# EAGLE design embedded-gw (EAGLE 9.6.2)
AUTHOR: Neal Jackson; REV: B; TITLE: Embedded GW

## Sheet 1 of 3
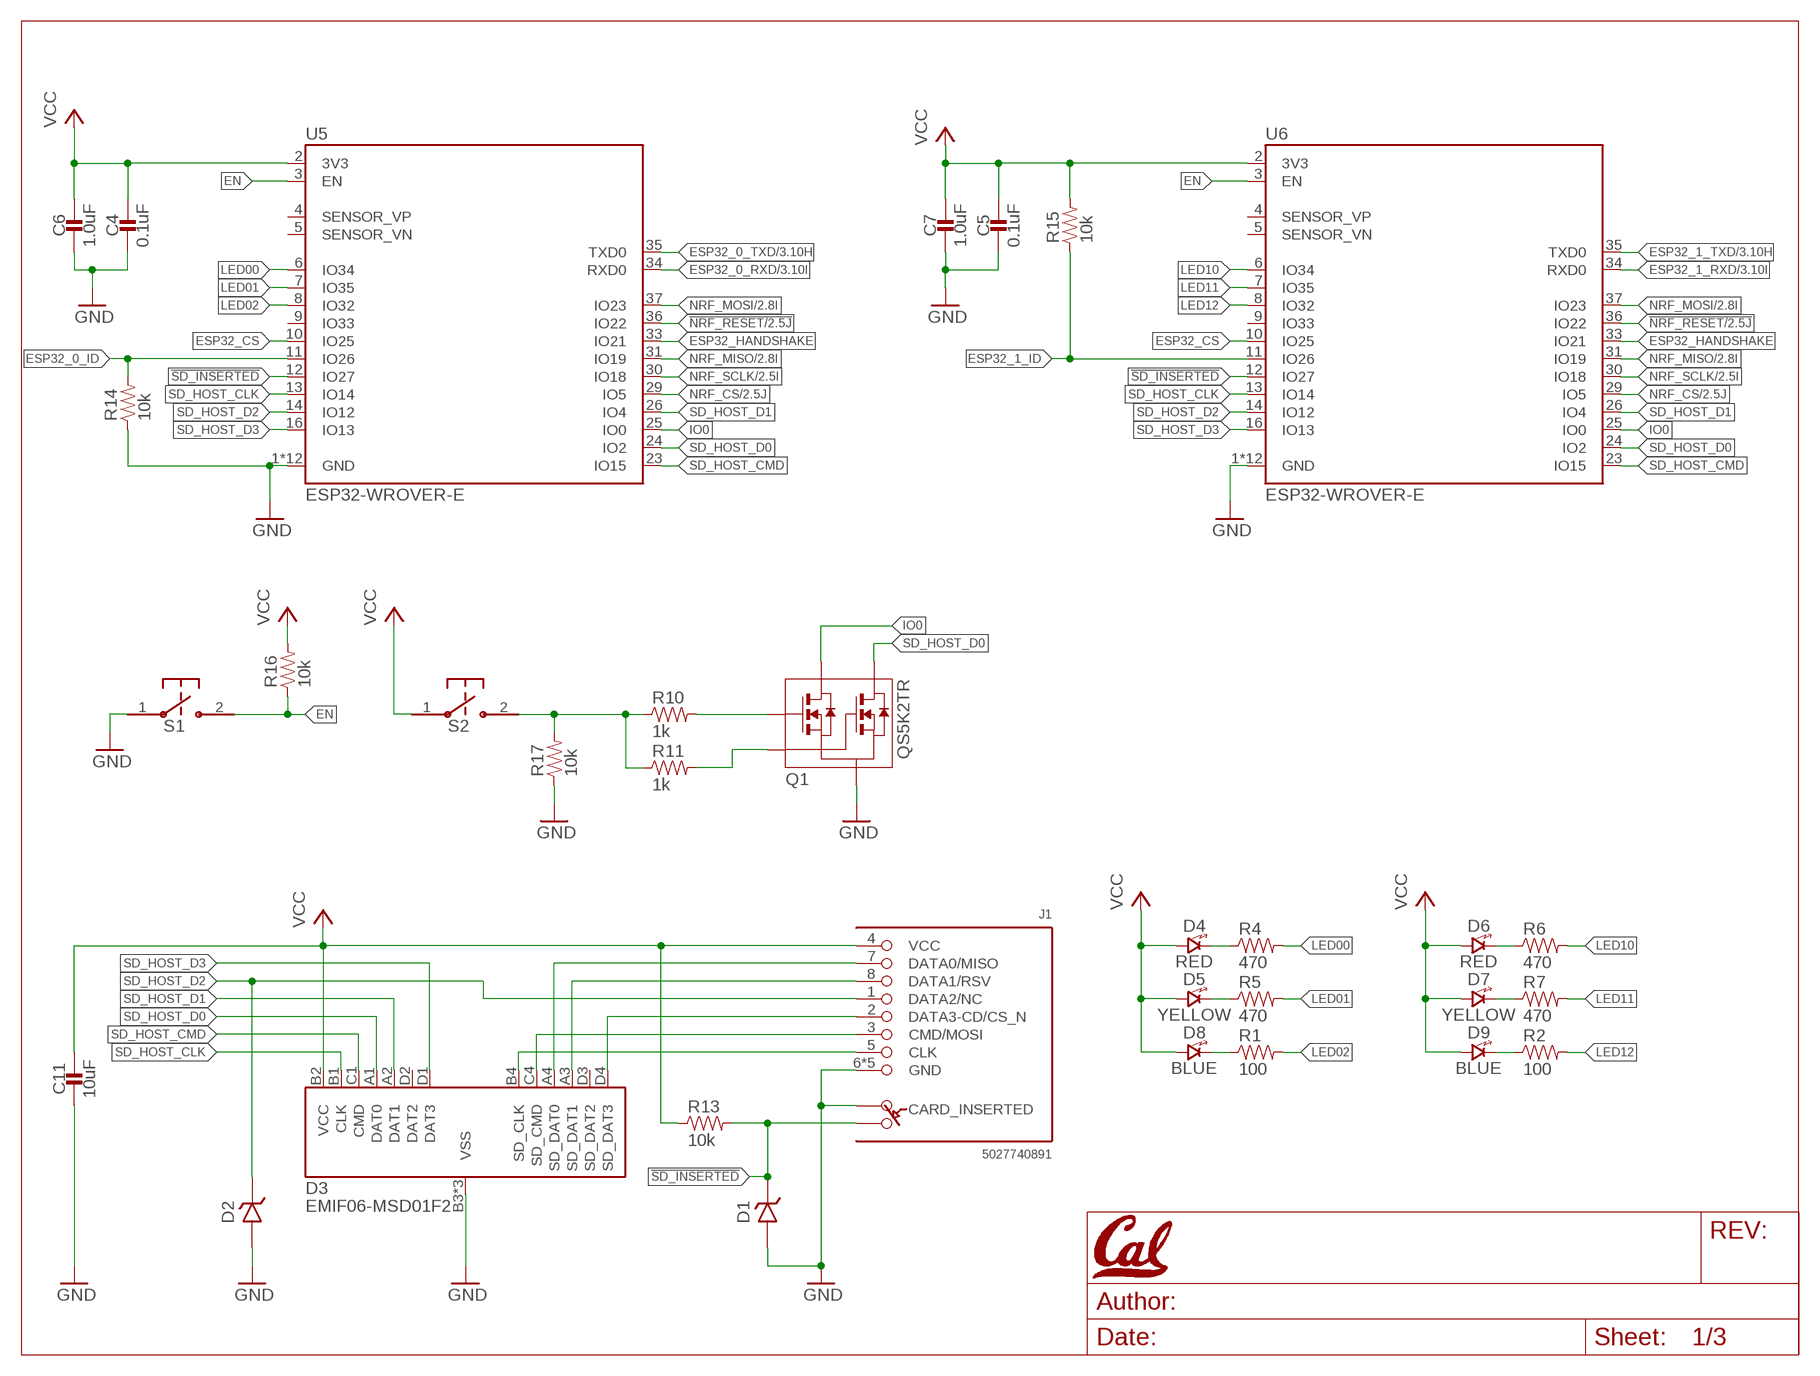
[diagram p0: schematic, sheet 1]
U$1 (LETTER_L_CAL): HEIGHT: 8.5in; WIDTH: 11in

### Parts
C4  0.1uF  CAPACITOR0402_CAP  [0402_CAP]
C5  0.1uF  CAPACITOR0402_CAP  [0402_CAP]
C6  1.0uF  CAPACITOR0402_CAP  [0402_CAP]
C7  1.0uF  CAPACITOR0402_CAP  [0402_CAP]
C11  10uF  CAPACITOR0805_CAP  [0805_CAP]
D1  DIODE_ZENER0201  [0201_DIODE]
D2  DIODE_ZENER0201  [0201_DIODE]
D3  EMIF06-MSD01F2  [BGA16C50P4X4_192X192X65N]
D4  RED  LED0603  [LED-0603]
D5  YELLOW  LED0603  [LED-0603]
D6  RED  LED0603  [LED-0603]
D7  YELLOW  LED0603  [LED-0603]
D8  BLUE  LED0603  [LED-0603]
D9  BLUE  LED0603  [LED-0603]
J1  5027740891  [5027740891]
Q1  QS5K2TR  [SOT95P280X100-5N]
R1  100  RESISTOR0402_RES  [0402_RES]
R2  100  RESISTOR0402_RES  [0402_RES]
R4  470  RESISTOR0402_RES  [0402_RES]
R5  470  RESISTOR0402_RES  [0402_RES]
R6  470  RESISTOR0402_RES  [0402_RES]
R7  470  RESISTOR0402_RES  [0402_RES]
R10  1k  RESISTOR0402_RES  [0402_RES]
R11  1k  RESISTOR0402_RES  [0402_RES]
R13  10k  RESISTOR0402_RES  [0402_RES]
R14  10k  RESISTOR0402_RES  [0402_RES]
R15  10k  RESISTOR0402_RES  [0402_RES]
R16  10k  RESISTOR0402_RES  [0402_RES]
R17  10k  RESISTOR0402_RES  [0402_RES]
S1  B3U-1000P  [B3U-1000P]
S2  B3U-1000P  [B3U-1000P]
U5  ESP32-WROVER-E  [ESP32-WROVER-E]
U6  ESP32-WROVER-E  [ESP32-WROVER-E]

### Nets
!NRF_RESET: U5.36(IO22) U6.36(IO22) ; also sheet 2
!SD_INSERTED: D1.P$1(CATHODE) J1.SWITCH(B) R13.2 U5.12(IO27) U6.12(IO27)
EN: R16.1 S1.2 U5.3(EN) U6.3(EN)
ESP32_0_ID: R14.2 U5.11(IO26)
ESP32_0_RXD: U5.34(RXD0) ; also sheet 3
ESP32_0_TXD: U5.35(TXD0) ; also sheet 3
ESP32_1_ID: R15.1 U6.11(IO26)
ESP32_1_RXD: U6.34(RXD0) ; also sheet 3
ESP32_1_TXD: U6.35(TXD0) ; also sheet 3
ESP32_CS: U5.10(IO25) U6.10(IO25)
ESP32_HANDSHAKE: U5.33(IO21) U6.33(IO21)
GND: C4.2 C5.2 C6.2 C7.2 C11.P$2 D1.P$2(ANODE) D2.P$2(ANODE) D3.B3(VSS) D3.C2(VSS) D3.C3(VSS) J1.6(GND) J1.DETECT(A) J1.GND1(GND) J1.GND2(GND) J1.GND3(GND) J1.GND4(GND) Q1.2(S) R14.1 R17.1 S1.1 U5.1(GND) U5.15(GND) U5.38(GND) U5.GND1(GND) U5.GND2(GND) U5.GND3(GND) U5.GND4(GND) U5.GND5(GND) U5.GND6(GND) U5.GND7(GND) U5.GND8(GND) U5.GND9(GND) U6.1(GND) U6.15(GND) U6.38(GND) U6.GND1(GND) U6.GND2(GND) U6.GND3(GND) U6.GND4(GND) U6.GND5(GND) U6.GND6(GND) U6.GND7(GND) U6.GND8(GND) U6.GND9(GND) ; also sheet 2,3
IO0: Q1.5(D1) U5.25(IO0) U6.25(IO0)
LED00: R4.2 U5.6(IO34)
LED01: R5.2 U5.7(IO35)
LED02: R1.2 U5.8(IO32)
LED10: R6.2 U6.6(IO34)
LED11: R7.2 U6.7(IO35)
LED12: R2.2 U6.8(IO32)
N$1: Q1.1(G1) R10.2
N$4: Q1.3(G2) R11.2
N$5: R10.1 R11.1 R17.2 S2.2
N$6: D3.C4(SD_CMD) J1.3(CMD/MOSI)
N$8: D3.A4(SD_DAT0) J1.7(DATA0/MISO)
N$9: D3.A3(SD_DAT1) J1.8(DATA1/RSV)
N$11: D3.D4(SD_DAT3) J1.2(DATA3-CD/CS_N)
N$12: D4.C(CATHODE) R4.1
N$13: D3.B4(SD_CLK) J1.5(CLK)
N$14: D5.C(CATHODE) R5.1
N$15: D8.C(CATHODE) R1.1
N$19: D6.C(CATHODE) R6.1
N$20: D7.C(CATHODE) R7.1
N$21: D9.C(CATHODE) R2.1
NRF_CS: U5.29(IO5) U6.29(IO5) ; also sheet 2
NRF_MISO: U5.31(IO19) U6.31(IO19) ; also sheet 2
NRF_MOSI: U5.37(IO23) U6.37(IO23) ; also sheet 2
NRF_SCLK: U5.30(IO18) U6.30(IO18) ; also sheet 2
SD_HOST_CLK: D3.B1(CLK) U5.13(IO14) U6.13(IO14)
SD_HOST_CMD: D3.C1(CMD) U5.23(IO15) U6.23(IO15)
SD_HOST_D0: D3.A1(DAT0) Q1.4(D2) U5.24(IO2) U6.24(IO2)
SD_HOST_D1: D3.A2(DAT1) U5.26(IO4) U6.26(IO4)
SD_HOST_D2: D2.P$1(CATHODE) J1.1(DATA2/NC) U5.14(IO12) U6.14(IO12)
SD_HOST_D3: D3.D1(DAT3) U5.16(IO13) U6.16(IO13)
VCC: C4.1 C5.1 C6.1 C7.1 C11.P$1 D3.B2(VCC) D4.A(ANODE) D5.A(ANODE) D6.A(ANODE) D7.A(ANODE) D8.A(ANODE) D9.A(ANODE) J1.4(VCC) R13.1 R15.2 R16.2 S2.1 U5.2(3V3) U6.2(3V3) ; also sheet 2,3
Unconnected: D3.D2(DAT2) D3.D3(SD_DAT2) U5.4(SENSOR_VP) U5.5(SENSOR_VN) U5.9(IO33) U6.4(SENSOR_VP) U6.5(SENSOR_VN) U6.9(IO33)

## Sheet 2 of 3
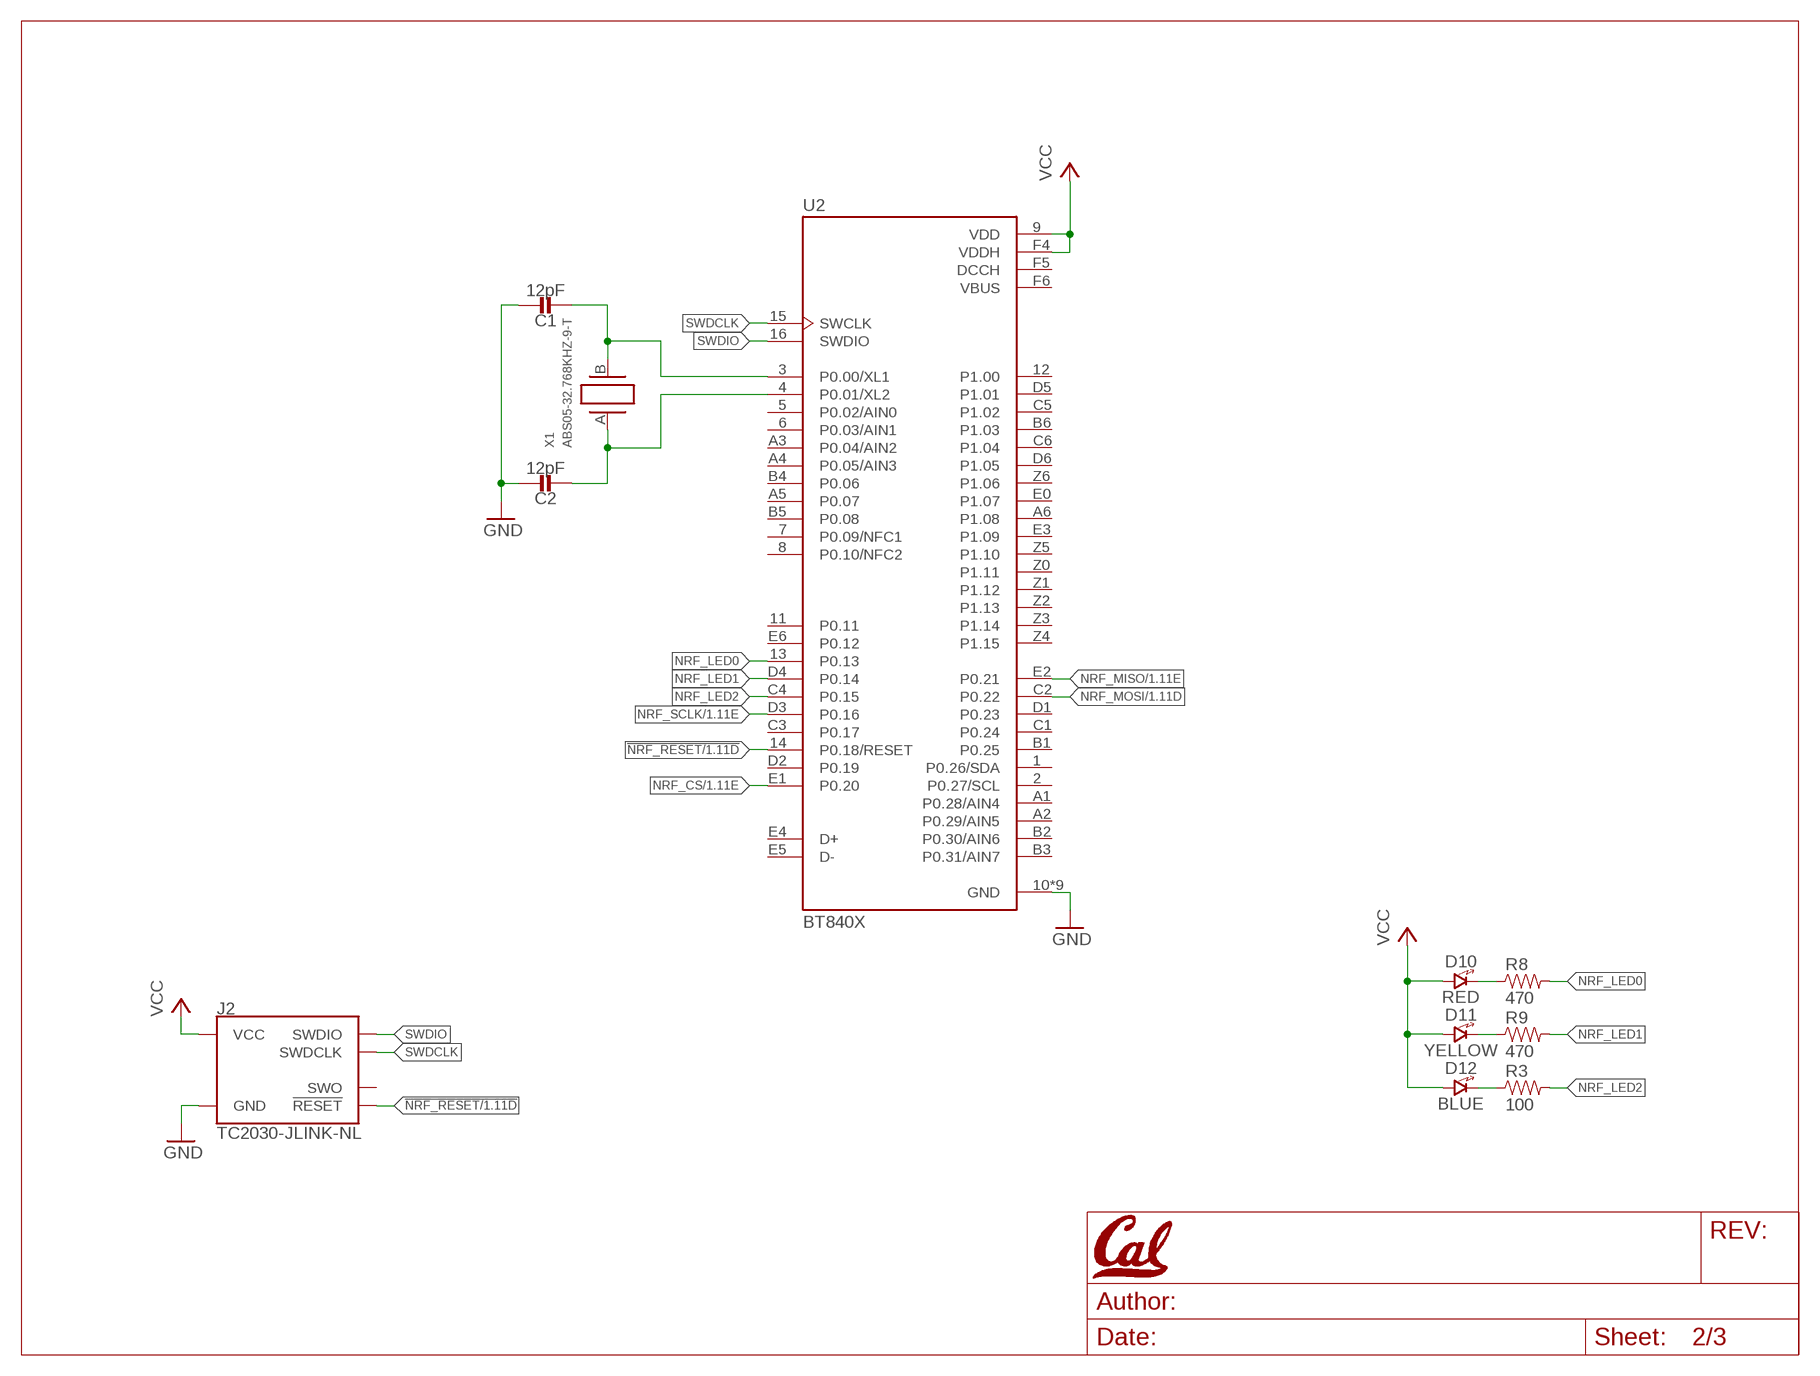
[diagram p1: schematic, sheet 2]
U$2 (LETTER_L_CAL): HEIGHT: 8.5in; WIDTH: 11in

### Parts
C1  12pF  CAPACITOR0402_CAP  [0402_CAP]
C2  12pF  CAPACITOR0402_CAP  [0402_CAP]
D10  RED  LED0603  [LED-0603]
D11  YELLOW  LED0603  [LED-0603]
D12  BLUE  LED0603  [LED-0603]
J2  TC2030-JLINK-NL  [TC2030-IDC-NL]
R3  100  RESISTOR0402_RES  [0402_RES]
R8  470  RESISTOR0402_RES  [0402_RES]
R9  470  RESISTOR0402_RES  [0402_RES]
U2  BT840X  [XCVR_BT840X]
X1  ABS05-32.768KHZ-9-T  [ABS05]

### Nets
!NRF_RESET: J2.3(!RESET) U2.14(P0.18/RESET) ; also sheet 1
GND: C1.1 C2.1 J2.5(GND) U2.10(GND) U2.A0(GND) U2.B0(GND) U2.C0(GND) U2.D0(GND) U2.F0(GND) U2.F1(GND) U2.F2(GND) U2.F3(GND) ; also sheet 1,3
N$2: C1.2 U2.3(P0.00/XL1) X1.B
N$3: C2.2 U2.4(P0.01/XL2) X1.A
N$22: D10.C(CATHODE) R8.1
N$23: D11.C(CATHODE) R9.1
N$24: D12.C(CATHODE) R3.1
NC: U2.F6(VBUS)
NRF_CS: U2.E1(P0.20) ; also sheet 1
NRF_LED0: R8.2 U2.13(P0.13)
NRF_LED1: R9.2 U2.D4(P0.14)
NRF_LED2: R3.2 U2.C4(P0.15)
NRF_MISO: U2.E2(P0.21) ; also sheet 1
NRF_MOSI: U2.C2(P0.22) ; also sheet 1
NRF_SCLK: U2.D3(P0.16) ; also sheet 1
SWDCLK: J2.4(SWDCLK) U2.15(SWCLK)
SWDIO: J2.2(SWDIO) U2.16(SWDIO)
VCC: D10.A(ANODE) D11.A(ANODE) D12.A(ANODE) J2.1(VCC) U2.9(VDD) U2.F4(VDDH) ; also sheet 1,3
Unconnected: J2.6(SWO) U2.1(P0.26/SDA) U2.2(P0.27/SCL) U2.5(P0.02/AIN0) U2.6(P0.03/AIN1) U2.7(P0.09/NFC1) U2.8(P0.10/NFC2) U2.11(P0.11) U2.12(P1.00) U2.A1(P0.28/AIN4) U2.A2(P0.29/AIN5) U2.A3(P0.04/AIN2) U2.A4(P0.05/AIN3) U2.A5(P0.07) U2.A6(P1.08) U2.B1(P0.25) U2.B2(P0.30/AIN6) U2.B3(P0.31/AIN7) U2.B4(P0.06) U2.B5(P0.08) U2.B6(P1.03) U2.C1(P0.24) U2.C3(P0.17) U2.C5(P1.02) U2.C6(P1.04) U2.D1(P0.23) U2.D2(P0.19) U2.D5(P1.01) U2.D6(P1.05) U2.E0(P1.07) U2.E3(P1.09) U2.E4(D+) U2.E5(D-) U2.E6(P0.12) U2.Z0(P1.11) U2.Z1(P1.12) U2.Z2(P1.13) U2.Z3(P1.14) U2.Z4(P1.15) U2.Z5(P1.10) U2.Z6(P1.06)

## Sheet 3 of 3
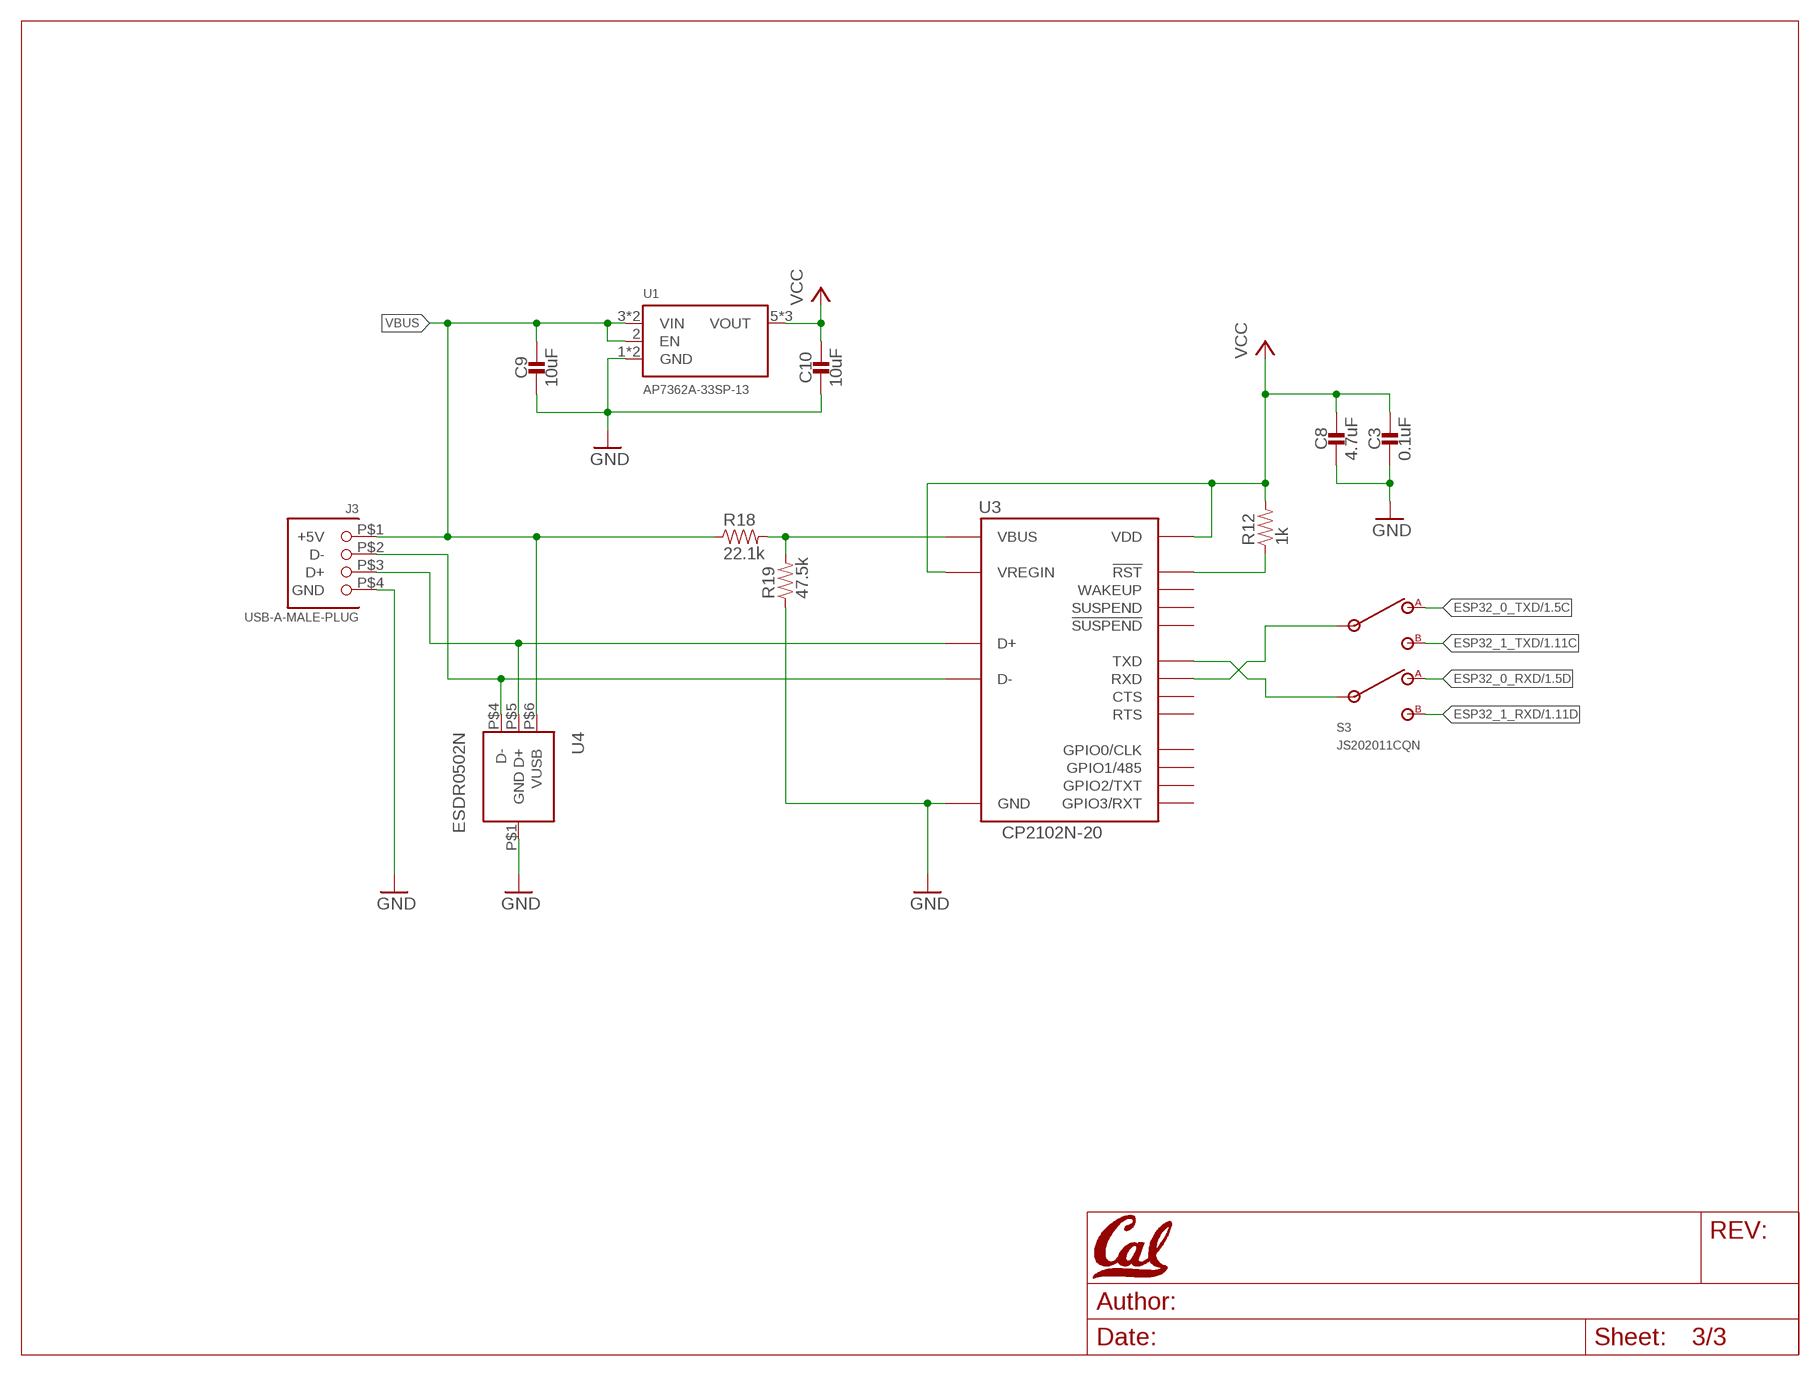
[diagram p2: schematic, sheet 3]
U$3 (LETTER_L_CAL): HEIGHT: 8.5in; WIDTH: 11in

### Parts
C3  0.1uF  CAPACITOR0402_CAP  [0402_CAP]
C8  4.7uF  CAPACITOR0603_CAP  [0603_CAP]
C9  10uF  CAPACITOR0805_CAP  [0805_CAP]
C10  10uF  CAPACITOR0805_CAP  [0805_CAP]
J3  USB-A-MALE-PLUG  [USB_A_MALE_PLUG_CUI_UP2-AH]
R12  1k  RESISTOR0402_RES  [0402_RES]
R18  22.1k  RESISTOR0402_RES  [0402_RES]
R19  47.5k  RESISTOR0402_RES  [0402_RES]
S3  JS202011CQN  [JS202011CQN]
U1  AP7362A-33SP-13  [SO-8EP]
U3  CP2102N-20  [QFN-20-3MM]
U4  ESDR0502N  [UDFN-6]

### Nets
D+: J3.P$3(D+) U3.4(D+) U4.P$5(D+)
D-: J3.P$2(D-) U3.5(D-) U4.P$4(D-)
ESP32_0_RXD: S3.1(A2) ; also sheet 1
ESP32_0_TXD: S3.4(A1) ; also sheet 1
ESP32_1_RXD: S3.3(B2) ; also sheet 1
ESP32_1_TXD: S3.6(B1) ; also sheet 1
GND: C3.2 C8.2 C9.P$2 C10.P$2 J3.P$4(GND) R19.1 U1.1(GND) U1.PAD(GND) U3.3(GND) U3.12(GND) U3.P$1(GND) U4.P$1(GND) ; also sheet 1,2
N$7: R12.1 U3.9(!RST)
N$10: R18.2 R19.2 U3.8(VBUS)
RXD: S3.2(I2) U3.18(TXD)
TXD: S3.5(I1) U3.17(RXD)
VBUS: C9.P$1 J3.P$1(+5V) R18.1 U1.2(EN) U1.3(VIN) U1.4(VIN) U4.P$6(VUSB)
VCC: C3.1 C8.1 C10.P$1 R12.2 U1.5(VOUT) U1.6(VOUT) U1.7(VOUT) U3.6(VDD) U3.7(VREGIN) ; also sheet 1,2
Unconnected: U3.1(GPIO1/485) U3.2(GPIO0/CLK) U3.11(!SUSPEND) U3.13(WAKEUP) U3.14(SUSPEND) U3.15(CTS) U3.16(RTS) U3.19(GPIO3/RXT) U3.20(GPIO2/TXT)

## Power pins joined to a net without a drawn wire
DCCH: U2.F5(DCCH)

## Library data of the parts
C1 C2 = passives:CAPACITOR: SMD Capacitor; DIGIKEY: 490-GCM1555C1H120GA16DCT-ND; MPN: GCM1555C1H120GA16D
C3-C5 = passives:CAPACITOR: SMD Capacitor; DIGIKEY: 1276-1511-1-ND; MPN: CL05B104KQ5NNNC
C6 C7 = passives:CAPACITOR: SMD Capacitor; DIGIKEY: 1276-1010-1-ND; MPN: CL05A105KQ5NNNC
C8 = passives:CAPACITOR: SMD Capacitor; DIGIKEY: 1276-1045-1-ND; MPN: CL10A475KQ8NNNC
C9-C11 = passives:CAPACITOR: SMD Capacitor; DIGIKEY: 1276-2404-1-ND; MPN: CL21A106KQCLNNC
D1 D2 = passives:DIODE_ZENER; DIGIKEY: ESD7381MUT5GOSCT-ND; MPN: ESD7381MUT5G
D3 = passives:EMIF06-MSD01F2: Mini and micro SD Card - EMI filtering and 25 kV ESD protection; DIGIKEY: 497-5903-1-ND; MANUFACTURER: STMicroelectronics; MOUSER: 511-EMIF06-MSD01F2; MPN: EMIF06-MSD01F2
D4 D6 D10 = leds:LED: LED; DIGIKEY: 160-1830-1-ND; MPN: LTST-C193KRKT-5A
D5 D7 D11 = leds:LED: LED; DIGIKEY: 160-1831-1-ND; MPN: LTST-C193KSKT-5A
D8 D9 D12 = leds:LED: LED; DIGIKEY: 160-1827-1-ND; MPN: LTST-C193TBKT-5A
J1 = connector:5027740891: CONN MICRO SD CARD PUSH-PUSH R/A; DIGIKEY: WM24066CT-ND; MANUFACTURER: Molex; MPN: 5027740891
J2 = connector:TC2030-JLINK
J3 = connector:USB-A-MALE-PLUG: USB A Male plug connector; DIGIKEY: 102-3996-ND; MANUFACTURER: CUI; MPN: UP2-AH-1-TH
Q1 = fets:QS5K2TR: 2.5V Drive Nch+Nch MOSFET; DIGIKEY: QS5K2CT-ND; MANUFACTURER: Rohm; MPN: QS5K2TR
R1-R3 = passives:RESISTOR: Resistor; DIGIKEY: 311-100JRCT-ND; MPN: RC0402JR-07100RL
R4-R9 = passives:RESISTOR: Resistor; DIGIKEY: 311-470LRCT-ND; MPN: RC0402FR-07470RL
R10-R12 = passives:RESISTOR: Resistor; DIGIKEY: RMCF0402JT1K00CT-ND; MPN: RMCF0402JT1K00
R13-R17 = passives:RESISTOR: Resistor; DIGIKEY: RMCF0402JT10K0CT-ND; MPN: RMCF0402JT10K0
R18 = passives:RESISTOR: Resistor; DIGIKEY: 311-22.1KLRCT-ND; MPN: RC0402FR-0722K1L
R19 = passives:RESISTOR: Resistor; DIGIKEY: 13-RT0402FRE0722K1LCT-ND; MPN: RT0402FRE0722K1L
S1 S2 = switches:B3U: Switch; DIGIKEY: SW1020CT-ND; MANUFACTURER: Omron; MPN: B3U-1000P
S3 = switches:JS202011CQN: DPDT through hole; DIGIKEY: 401-2001-ND; MANUFACTURER: C&K; MPN: JS202011CQN
U1 = chips:AP7362: The AP7362 is a 1.5A adjustable/fixed output voltage linear regulator with ultra-low dropout; DIGIKEY: AP7362A-33SP-13DICT-ND; MANUFACTURER: Diodes Incorporated; MPN: AP7362A-33SP-13
U2 = BT840X:BT840X: 802.15.4, Bluetooth Bluetooth v5.0, Thread, Zigbee® Transceiver Module 2.4GHz PCB Trace Surface Mou Check prices; DIGIKEY: 1914-BT840XCT-ND; MANUFACTURER: Fanstel Corp.; MPN: BT840X
U3 = chips:CP2102N-20: A cheap, simple USB to UART adapter; DIGIKEY: 336-5885-ND; MANUFACTURER: SiLabs; MPN: CP2102N-A02-GQFN20
U4 = chips:ESDR0502N; DIGIKEY: ESDR0502NMUTBGOSCT-ND; MPN: ESDR0502NMUTBG
U5 U6 = chips:ESP32-WROVER-E; DIGIKEY: 1965-ESP32-WROVER-E(8MB)CT-ND; MANUFACTURER: Espressif Systems; MPN: ESP32-WROVER-E (8MB)
X1 = crystals:ABS05-32.768KHZ: 32.768kHz Crystal; DIGIKEY: 535-11897-1-ND; MANUFACTURER: Abracon; MPN: ABS05-32.768KHZ-9-T

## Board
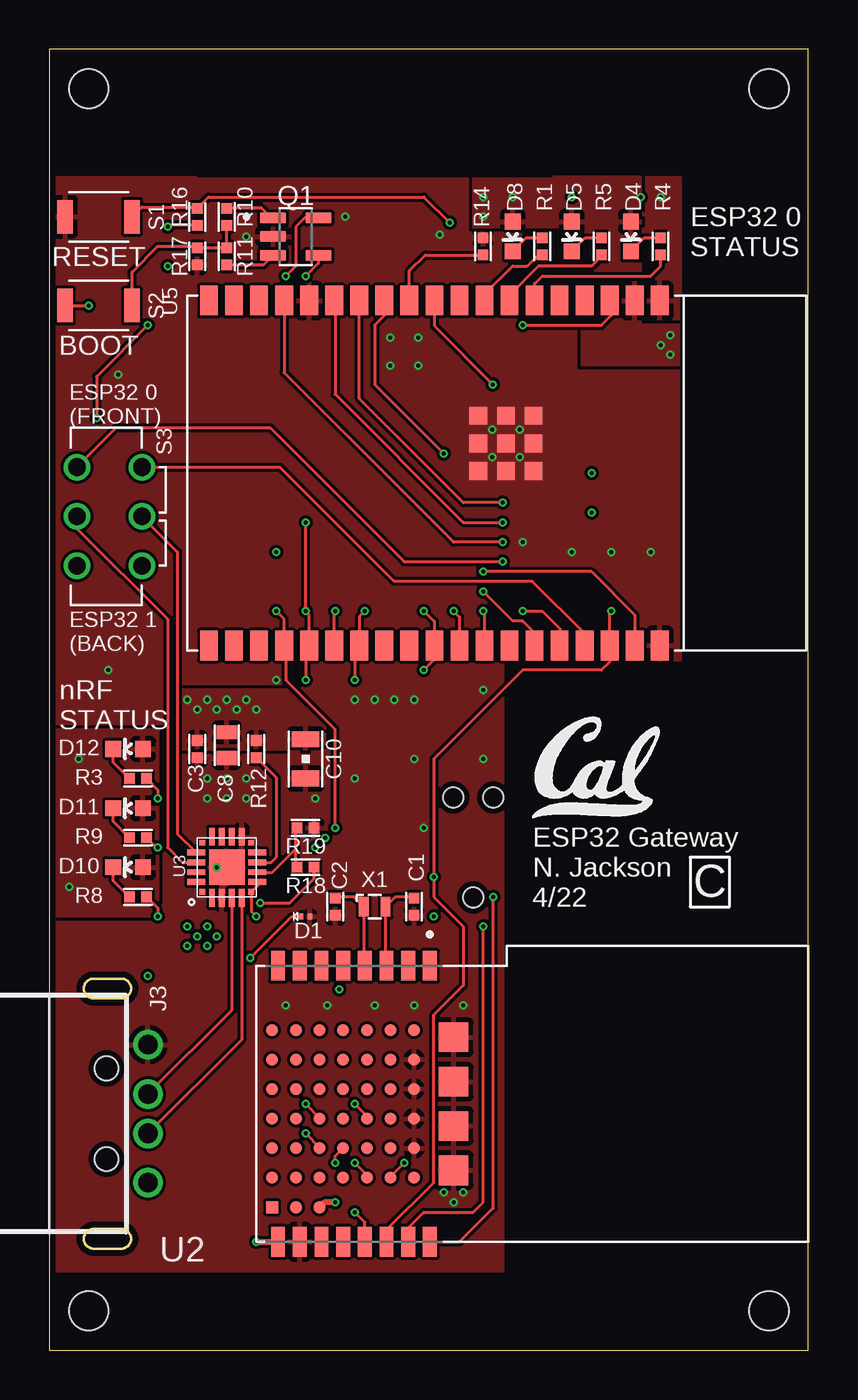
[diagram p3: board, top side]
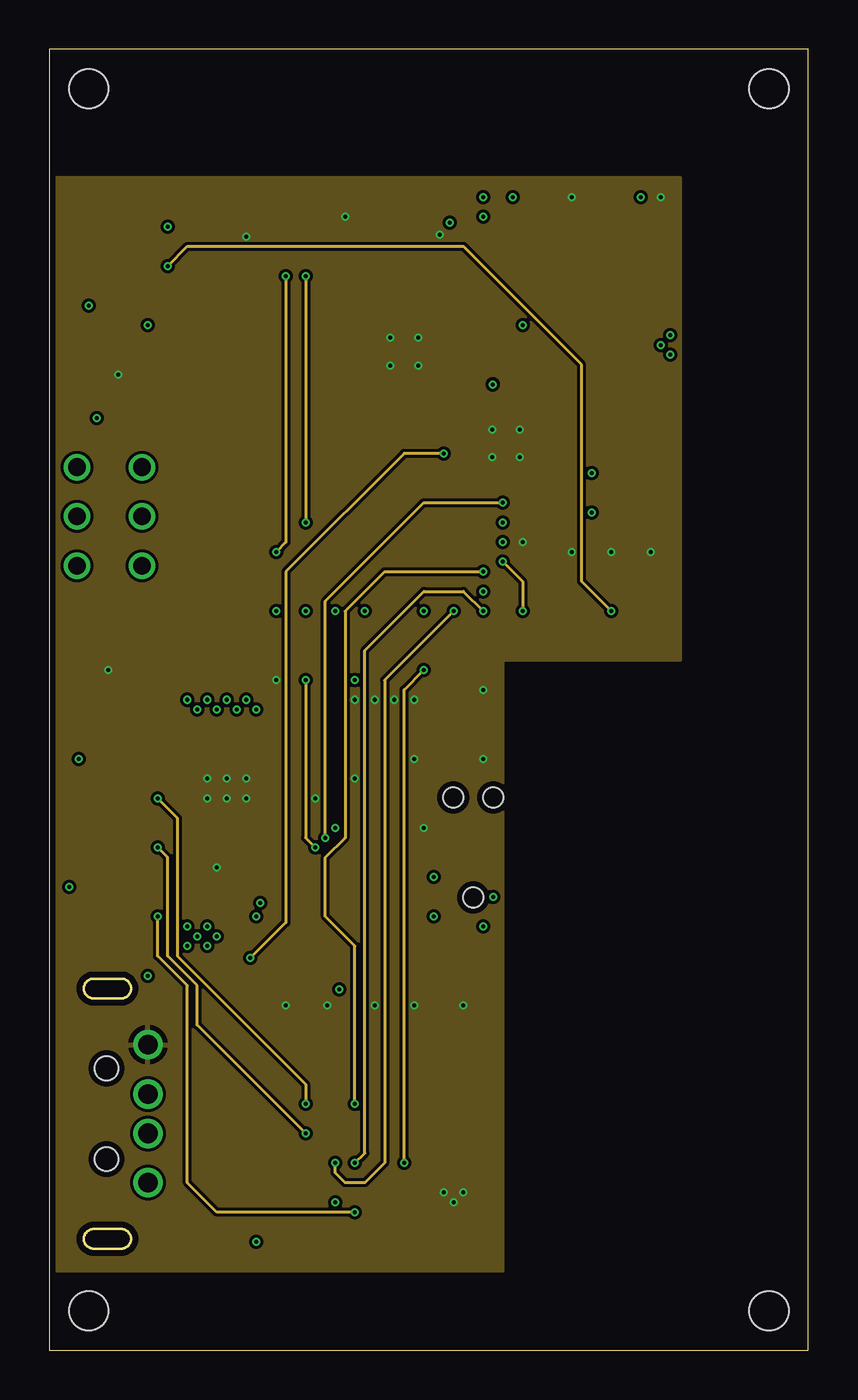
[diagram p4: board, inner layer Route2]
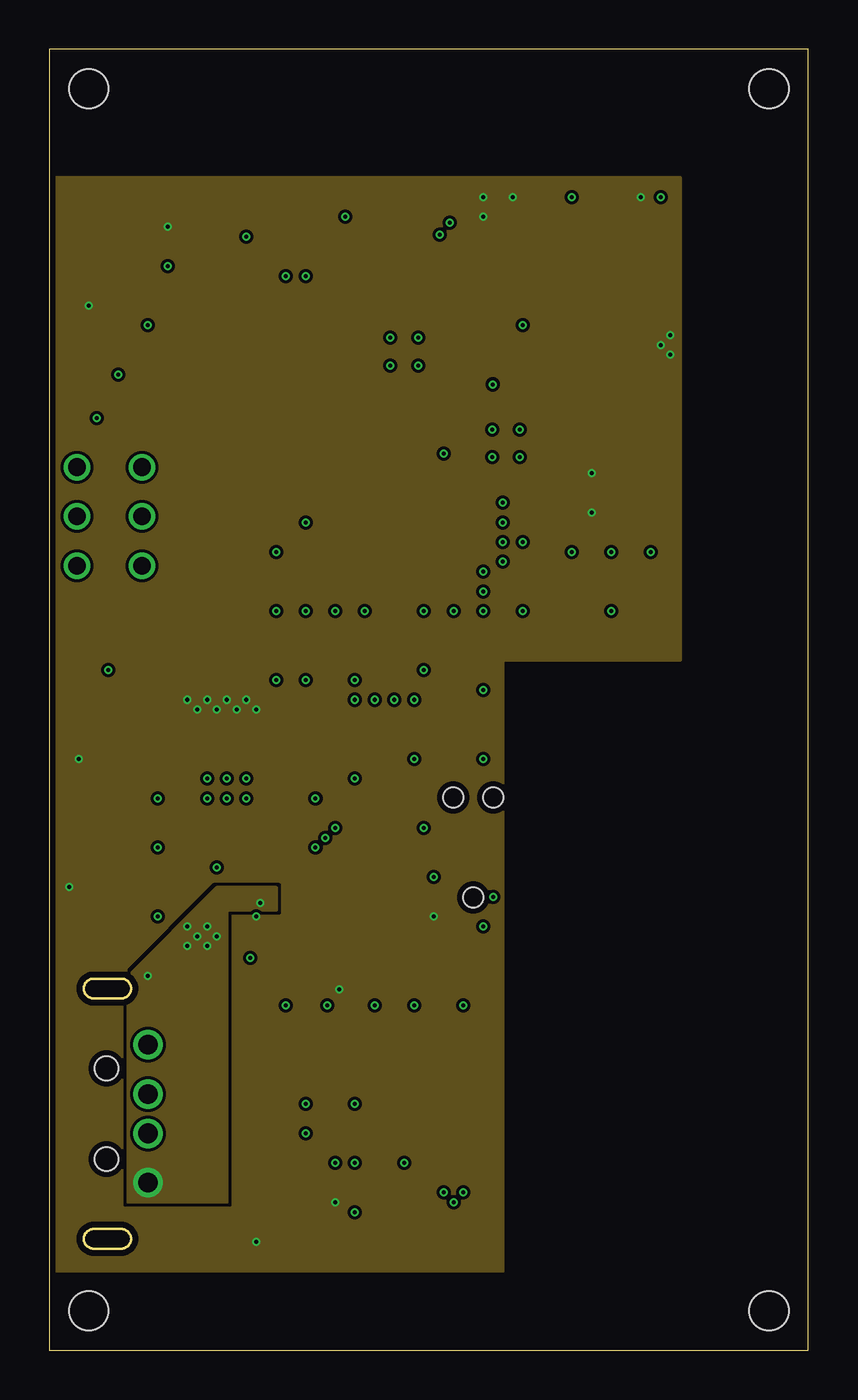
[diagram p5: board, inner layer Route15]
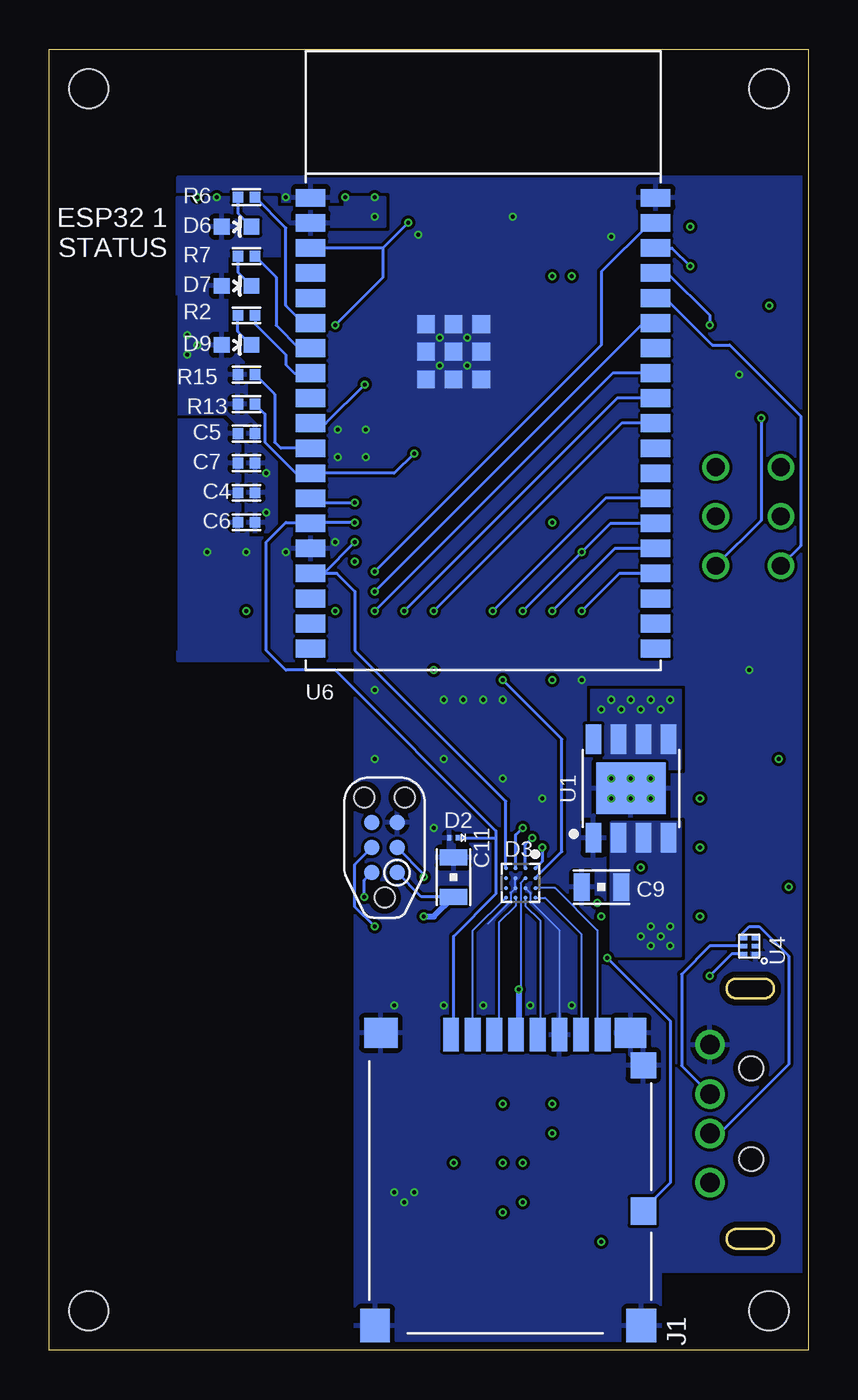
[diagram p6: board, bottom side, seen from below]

Size 38.5 x 66 mm. Coordinates in mm from the lower left corner, seen from the top.
Outline: 0,0 38.5,0 38.5,66 0,66 0,0
Copper layers (1+2*15+16): Top 0.018mm / dielectric 0.25mm / Route2 0.035mm / dielectric 1.024mm / Route15 0.035mm / dielectric 0.25mm / Bottom 0.018mm
Design rules "quickturn_co_kr_1oz_4lyr *": minimum track width 4mil, minimum drill 8mil, track to track 6mil, track to pad 6mil, pad to pad 6mil, via to via 6mil, smd to smd 6mil, copper to edge 12mil, drill to drill 12mil, minimum pad ring 8mil, minimum via ring 4mil, stop-mask expansion 3mil, vias tented up to drill 50mil, thermal gap 10mil
Holes 2 mm at 2,64 36.5,64 2,2 36.5,2

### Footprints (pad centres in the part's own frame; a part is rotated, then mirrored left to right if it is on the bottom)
0402_CAP = smd 0.536 x 0.546: 1 -0.433,0; 2 0.433,0
0603_CAP = smd 0.7 x 1: 1 -0.65,0; 2 0.65,0
0805_CAP = smd 0.8 x 1.4: P$1 1,0; P$2 -1,0
0201_DIODE = smd 0.3 x 0.21: P$1 0,0.22; P$2 0,-0.22
BGA16C50P4X4_192X192X65N = smd 0.2 x 0.2: A1 -0.75,0.75; A2 -0.25,0.75; A3 0.25,0.75; A4 0.75,0.75; B1 -0.75,0.25; B2 -0.25,0.25; B3 0.25,0.25; B4 0.75,0.25; C1 -0.75,-0.25; C2 -0.25,-0.25; C3 0.25,-0.25; C4 0.75,-0.25; D1 -0.75,-0.75; D2 -0.25,-0.75; D3 0.25,-0.75; D4 0.75,-0.75
LED-0603 = smd 0.8 x 0.8: A 0,-0.75; C 0,0.75
5027740891 = smd 0.8 x 1.68: 1 3.3,0.84; 2 2.2,0.84; 3 1.1,0.84; 4 0,0.84; 5 -1.1,0.84; 6 -2.2,0.84; 7 -3.3,0.84; 8 -4.4,0.84 | smd 1.29 x 1.3: DETECT -6.455,2.4 | smd 1.7 x 1.5: GND1 6.85,0.75 | smd 1.6 x 1.5: GND2 -5.81,0.75 | smd 1.5 x 1.7: GND3 -6.35,15.6; GND4 7.15,15.6 | smd 1.29 x 1.4: SWITCH -6.455,9.8
TC2030-IDC-NL = smd 0.787 x 0.787: 1 -1.27,-0.635; 2 -1.27,0.635; 3 0,-0.635; 4 0,0.635; 5 1.27,-0.635; 6 1.27,0.635 | hole 1.016: -2.54,0; 2.54,1.016; 2.54,-1.016
USB_A_MALE_PLUG_CUI_UP2-AH = drill 1: P$1 3.5,5; P$2 1,5; P$3 -1,5; P$4 -3.5,5 | hole 1.2: -2.3,2.9; 2.3,2.9
SOT95P280X100-5N = smd 1.32 x 0.57: 1 -1.145,0.95; 2 -1.145,0; 3 -1.145,-0.95; 4 1.145,-0.95; 5 1.145,0.95
0402_RES = smd 0.536 x 0.546: 1 -0.433,0; 2 0.433,0
B3U-1000P = smd 0.8 x 1.7: 1 -1.7,0; 2 1.7,0
JS202011CQN = drill 0.9: 1 0,0; 2 2.5,0; 3 5,0; 4 0,3.3; 5 2.5,3.3; 6 5,3.3
SO-8EP = smd 1.505 x 0.802: 1 -2.5,1.905; 2 -2.5,0.635; 3 -2.5,-0.635; 4 -2.5,-1.905; 5 2.5,0.635; 6 2.5,-0.635; 7 2.5,-1.905; 8 2.5,1.905 | smd 2.613 x 3.502: PAD 0,0
XCVR_BT840X = smd 1.5 x 0.7: 1 -7,-5.2; 2 -7,-6.3; 3 -7,-7.4; 4 -7,-8.5; 5 -7,-9.6; 6 -7,-10.7; 7 -7,-11.8; 8 -7,-12.9; 9 7,-12.9; 10 7,-11.8; 11 7,-10.7; 12 7,-9.6; 13 7,-8.5; 14 7,-7.4; 15 7,-6.3; 16 7,-5.2 | smd 0.6 x 0.6: A0 -2.25,-6; A1 -2.25,-7.2; A2 -2.25,-8.4; A3 -2.25,-9.6; A4 -2.25,-10.8; A5 -2.25,-12; A6 -2.25,-13.2; B0 -0.75,-6; B1 -0.75,-7.2; B2 -0.75,-8.4; B3 -0.75,-9.6; B4 -0.75,-10.8; B5 -0.75,-12; B6 -0.75,-13.2; C0 0.75,-6; C1 0.75,-7.2; C2 0.75,-8.4; C3 0.75,-9.6; C4 0.75,-10.8; C5 0.75,-12; C6 0.75,-13.2; D0 2.25,-6; D1 2.25,-7.2; D2 2.25,-8.4; D3 2.25,-9.6; D4 2.25,-10.8; D5 2.25,-12; D6 2.25,-13.2; E0 3.75,-6; E1 3.75,-7.2; E2 3.75,-8.4; E3 3.75,-9.6; E4 3.75,-10.8; E5 3.75,-12; E6 3.75,-13.2; F4 5.25,-10.8; F5 5.25,-12; F6 5.25,-13.2; Z0 -3.75,-6; Z1 -3.75,-7.2; Z2 -3.75,-8.4; Z3 -3.75,-9.6; Z4 -3.75,-10.8; Z5 -3.75,-12; Z6 -3.75,-13.2 | smd 1.5 x 1.5: F0 -3.375,-4; F1 -1.125,-4; F2 1.125,-4; F3 3.375,-4
QFN-20-3MM = smd 0.3 x 0.3: 1 -1.25,1.25; 6 -1.25,-1.25; 11 1.25,-1.25; 16 1.25,1.25 | smd 0.9 x 0.3: 2 -1.55,0.75; 3 -1.55,0.25; 4 -1.55,-0.25; 5 -1.55,-0.75; 12 1.55,-0.75; 13 1.55,-0.25; 14 1.55,0.25; 15 1.55,0.75 | smd 0.3 x 0.9: 7 -0.75,-1.55; 8 -0.25,-1.55; 9 0.25,-1.55; 10 0.75,-1.55; 17 0.75,1.55; 18 0.25,1.55; 19 -0.25,1.55; 20 -0.75,1.55 | smd 1.8 x 1.8: P$1 0,0
UDFN-6 = smd 0.42 x 0.22: P$1 -0.325,0.4; P$2 -0.325,0; P$3 -0.325,-0.4; P$4 0.325,-0.4; P$5 0.325,0; P$6 0.325,0.4
ESP32-WROVER-E = smd 1.5 x 0.9: 1 0.25,23.96; 2 0.25,22.69; 3 0.25,21.42; 4 0.25,20.15; 5 0.25,18.88; 6 0.25,17.61; 7 0.25,16.34; 8 0.25,15.07; 9 0.25,13.8; 10 0.25,12.53; 11 0.25,11.26; 12 0.25,9.99; 13 0.25,8.72; 14 0.25,7.45; 15 0.25,6.18; 16 0.25,4.91; 17 0.25,3.64; 18 0.25,2.37; 19 0.25,1.1; 20 17.75,1.1; 21 17.75,2.37; 22 17.75,3.64; 23 17.75,4.91; 24 17.75,6.18; 25 17.75,7.45; 26 17.75,8.72; 27 17.75,9.99; 28 17.75,11.26; 29 17.75,12.53; 30 17.75,13.8; 31 17.75,15.07; 32 17.75,16.34; 33 17.75,17.61; 34 17.75,18.88; 35 17.75,20.15; 36 17.75,21.42; 37 17.75,22.69; 38 17.75,23.96 | smd 0.9 x 0.9: GND1 6.1,17.56; GND2 7.5,17.56; GND3 8.9,17.56; GND4 6.1,16.16; GND5 7.5,16.16; GND6 8.9,16.16; GND7 6.1,14.76; GND8 7.5,14.76; GND9 8.9,14.76
ABS05 = smd 0.5 x 1: A -0.55,0; B 0.55,0

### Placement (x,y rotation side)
C1  18.5,22.5 90 top
C2  14.5,22.5 90 top
C3  7.5,30.5 270 top
C4  28.5,43.5 180 bottom
C5  28.5,46.5 180 bottom
C6  28.5,42 180 bottom
C7  28.5,45 180 bottom
C8  9,30.7 270 top
C9  10.5,23.5 0 bottom
C10  13,30 90 top
C11  18,24 270 bottom
D1  13,22 90 top
D2  18,26 270 bottom
D3  14.6,23.7 270 bottom
D4  29.5,56.5 180 top
D5  26.5,56.5 180 top
D6  29,57 270 bottom
D7  29,54 270 bottom
D8  23.5,56.5 180 top
D9  29,51 270 bottom
D10  4,24.5 90 top
D11  4,27.5 90 top
D12  4,30.5 90 top
J1  14.83,16.85 180 bottom
J2  21.5,25.5 90 bottom
J3  0,12 270 top
Q1  12.5,56.5 0 top
R1  25,56 270 top
R2  28.5,52.5 0 bottom
R3  4.5,29 0 top
R4  31,56 270 top
R5  28,56 270 top
R6  28.5,58.5 0 bottom
R7  28.5,55.5 0 bottom
R8  4.5,23 0 top
R9  4.5,26 0 top
R10  9,57.5 90 top
R11  9,55.5 270 top
R12  10.5,30.5 90 top
R13  28.5,48 0 bottom
R14  22,56 270 top
R15  28.5,49.5 180 bottom
R16  7.5,57.5 270 top
R17  7.5,55.5 90 top
R18  13,24.5 180 top
R19  13,26.5 180 top
S1  2.5,57.5 0 top
S2  2.5,53 0 top
S3  1.4,44.8 270 top
U1  9,28.5 90 bottom
U2  24.5,12.5 270 top
U3  9,24.5 90 top
U4  3,20.5 180 bottom
U5  7,53.5 270 top
U6  25.5,34.5 0 bottom
U$4  [UCB_CAL_200MIL]  24.5,27 0 top
X1  16.5,22.5 0 top

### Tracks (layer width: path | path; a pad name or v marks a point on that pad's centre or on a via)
!NRF_RESET  (via drill 0.2)
  Top 0.152: v28.5,37.5 28.42,37.42 U5.36 28.42,34.92 28,34.5 24,34.5 19.5,30 v19.5,24 19.5,23 21,21.5 21,18.5 19.5,17 19.5,8.5 17.1,6.1 U2.14
  Route2 0.152: v6,55 7,56 21,56 27,50 27,39 v28.5,37.5
  Bottom 0.152: v19.5,24 19.5,24.14 J2.3 | U6.36 6.92,55.92 v6,55
!SD_INSERTED  (via drill 0.2)
  Top 0.152: U5.12 16.99,52.49 16.5,52 16.5,49 v20,45.5 | v10.2,19.9 12.3,22 D1.P$1
  Route2 0.152: v20,45.5 18,45.5 12,39.5 12,21.7 v10.2,19.9
  Bottom 0.152: v10.2,19.9 7,16.7 7,8.5 8.38,7.12 J1.SWITCH | v20,45.5 21.01,44.49 U6.12 25.99,44.49 27.57,46.07 27.57,47.5 R13.2
D+
  Top 0.152: U3.4 9.25,17.25 J3.P$3
  Bottom 0.152: U4.P$5 5,20.5 6.43,19.07 6.43,14.43 J3.P$3
D-
  Top 0.152: U3.5 9.75,15.75 J3.P$2
  Bottom 0.152: U4.P$4 3.33,21.18 3,21.5 2.5,21.5 1,20 1,14.5 4.5,11 J3.P$2
EN  (via drill 0.2)
  Top 0.102: 28.5,52.5 28.5,53.17 U5.3
  Top 0.152: S1.2 4.7,58 7.43,58 R16.1 8.07,58.5 19,58.5 v20.3,57.2 | v24,52 28,52 28.5,52.5
  Bottom 0.152: v20.3,57.2 21.58,55.92 | 21.58,55.92 U6.3 | v24,52 21.58,54.42 21.58,55.92
ESP32_0_ID
  Top 0.152: U5.11 18.26,54.76 19.07,55.57 R14.2
ESP32_0_RXD  (via drill 0.2)
  Top 0.152: v24,37.5 25,37.5 25.88,36.62 U5.34 | v23,40 18,40 11.2,46.8 3.4,46.8 S3.1
  Route2 0.152: v23,40 24,39 v24,37.5
ESP32_0_TXD
  Top 0.152: U5.35 27.15,36.35 24.5,39 17.5,39 11.7,44.8 S3.4
ESP32_1_ID
  Bottom 0.152: U6.11 26.76,45.76 27.07,46.07 27.07,48.5 R15.1
ESP32_1_RXD
  Bottom 0.152: U6.34 7.25,53.38 4.87,51 4,51 0.4,47.4 0.4,40.8 S3.3
ESP32_1_TXD  (via drill 0.2)
  Top 0.152: v5,52 2.4,49.4 v2.4,47.3
  Bottom 0.152: U6.35 7.15,54.65 5,52.5 v5,52 | v2.4,47.3 2.4,42.1 S3.6
ESP32_CS  (via drill 0.2)
  Top 0.152: U5.10 19.53,51.97 v22.5,49
  Bottom 0.152: U6.10 24.47,47.03 v22.5,49
ESP32_HANDSHAKE  (via drill 0.2)
  Top 0.152: v22,38.5 23.5,37 24,37 24.61,36.39 U5.33
  Bottom 0.152: U6.33 8.39,52.11 v22,38.5
GND  (via drill 0.2)
  Bottom 0.102: J1.6 12.63,16.72 12.61,16.74 12.61,21.3 14.1,22.8 14.1,23.2 D3.B3 | D3.C2 14.9,23.9 14.9,23.5 D3.C3 15.1,23.2 15.1,22.8 16.25,21.65
  other vias: 8,29 9,29 10,29 8,28 9,28 10,28 8.5,24.5 20,8 21,8 20.5,7.5 21,17.5 18.5,17.5 11.5,34 17.3,51.36 18.7,51.36 17.3,49.96 18.7,49.96 22.46,46.7 23.86,46.7 22.46,45.3 23.86,45.3 13.5,28 31,58.5 26.5,58.5 14.1,17.5 19,26.5 22,30 15.5,29 26.5,40.5 24,41 28.5,40.5 30.5,40.5 22,33.5 18.5,30 18.5,33 17.5,33 16.5,33 15.5,33 12,17.5 10,56.5 16.5,17.5 3,34.5 3.5,49.5 15,57.5 19.8,56.6
  pour Top (rank 2): 0,59.5 32,59.5 32,35 23,35 23,4 0,4
  pour Bottom (rank 2): 0,59.5 32,59.5 32,35 23,35 23,0.5 7.5,0.5 7.5,4 0,4
  pour Route2: 0,59.5 32,59.5 32,35 23,35 23,4 0,4
  pour Bottom (no thermals): 15.5,53 15.5,48 20.5,48 20.5,53
  pour Top (no thermals): 20.5,48.5 25.5,48.5 25.5,43.5 20.5,43.5
IO0  (via drill 0.2)
  Top 0.152: U5.25 14.45,37.45 v14.5,37.5 | Q1.5 12.95,57.45 12.5,57 12.5,55 v12,54.5
  Route2 0.152: v12,54.5 12,41 v11.5,40.5
  Bottom 0.152: U6.25 10.05,41.95 v11.5,40.5 v14.5,37.5
LED00
  Top 0.152: U5.6 24.61,54.11 25,54.5 30.5,54.5 31,55 R4.2
LED01
  Top 0.152: R5.2 28,55.5 27.5,55 24.81,55 23.34,53.53 U5.7
LED02
  Top 0.152: U5.8 22.07,53.57 23.5,55 24.23,55 24.8,55.57 R1.2
LED10
  Bottom 0.152: U6.6 25.61,52.11 26.5,53 26.5,56.93 R6.2
LED11
  Bottom 0.152: R7.2 27,54.43 27,52 25.84,50.84 U6.7
LED12
  Bottom 0.152: R2.2 28.07,52.07 26.5,50.5 26.5,50 26.07,49.57 U6.8
N$1
  Top 0.152: R10.2 10.77,57.93 11.25,57.45 Q1.1
N$2
  Top 0.152: U2.3 17.05,19.55 X1.B 17.55,23 18.43,23 C1.2
N$3
  Top 0.152: C2.2 14.57,23 15.45,23 X1.A 15.95,19.55 U2.4
N$4
  Top 0.152: R11.2 10.5,55.07 10.77,55.07 10.87,55.07 Q1.3
N$5
  Top 0.152: S2.2 4.2,54.7 5.5,56 7.43,56 R17.2 R11.1 R10.1
N$6
  Bottom 0.102: J1.3 15.72,16.22 15.7,16.3 15.7,21.7 14.85,22.55 D3.C4
N$7
  Top 0.152: U3.9 11.25,24.75 11.5,25 11.5,29.07 R12.1
N$8
  Bottom 0.102: D3.A4 13.35,22.95 11.5,21.1 11.5,17.5 11.5,15.98 J1.7
N$9
  Bottom 0.102: D3.A3 12.85,23.45 10.7,21.3 10.7,16.28 J1.8
N$10
  Top 0.152: R19.2 12.5,26.43 12.5,25.5 12.5,25.43 | U3.8 11.32,24.25 12.5,25.43 | R18.2 12.5,24.57 12.5,25.43
N$11
  Bottom 0.102: J1.2 17.03,19.47 17.02,21.3 D3.D4
N$12
  Top 0.152: D4.C 30.18,56.43 R4.1
N$13
  Bottom 0.102: J1.5 13.6,16.14 13.6,21.8 14.35,22.55 D3.B4
N$14
  Top 0.152: D5.C 27.18,56.43 R5.1
N$15
  Top 0.152: D8.C 24.18,56.43 R1.1
N$19
  Bottom 0.152: R6.1 28.93,57.68 D6.C
N$20
  Bottom 0.152: R7.1 28.93,54.68 D7.C
N$21
  Bottom 0.152: D9.C 28.93,51.68 R2.1
N$22
  Top 0.152: R8.1 3.25,23.82 D10.C
N$23
  Top 0.152: R9.1 3.25,26.82 D11.C
N$24
  Top 0.152: R3.1 3.25,29.82 D12.C
NRF_CS  (via drill 0.2)
  Top 0.152: U2.E1 17.3,8.8 v18,9.5 | v19,37.5 19.53,36.97 U5.29 19.53,35.03 v19,34.5
  Route2 0.152: v19,34.5 18,33.5 v18,9.5
  Bottom 0.152: U6.29 9.47,47.03 v19,37.5
NRF_LED0  (via drill 0.2)
  Top 0.152: R8.2 5.5,22.43 v5.5,22 | U2.13 16,6.5 v15.5,7
  Route2 0.152: v15.5,7 8.5,7 7,8.5 7,18.5 5.5,20 v5.5,22
NRF_LED1  (via drill 0.2)
  Top 0.152: v13,11 13.7,10.3 U2.D4 | R9.2 5.43,25.5 v5.5,25.5
  Route2 0.152: v13,11 7.5,16.5 7.5,18.5 6,20 6,25 v5.5,25.5
NRF_LED2  (via drill 0.2)
  Top 0.152: v13,12.5 13.7,11.8 U2.C4 | R3.2 5.5,28.43 v5.5,28
  Route2 0.152: v5.5,28 6.5,27 6.5,20 13,13.5 v13,12.5
NRF_MISO  (via drill 0.2)
  Top 0.152: v15.5,9.5 16.1,8.9 U2.E2 | v22,37.5 22.07,37.43 U5.31
  Route2 0.152: v15.5,9.5 16,10 16,35.5 19,38.5 21,38.5 v22,37.5
  Bottom 0.152: U6.31 9.93,49.57 v22,37.5
NRF_MOSI  (via drill 0.2)
  Top 0.152: v15.5,12.5 16.1,11.9 U2.C2 | v22,39.5 27.5,39.5 29.69,37.31 U5.37
  Route2 0.152: v15.5,12.5 15.5,20.5 14,22 14,25 15,26 15,37.5 17,39.5 v22,39.5
  Bottom 0.152: U6.37 8.03,57.19 10.5,54.72 10.5,51 v22,39.5
NRF_SCLK  (via drill 0.2)
  Top 0.152: v20.5,37.5 20.8,37.2 U5.30 | v14.5,9.5 14.5,9.85 U2.D3
  Route2 0.152: v20.5,37.5 17,34 17,9.5 16,8.5 15,8.5 14.5,9 v14.5,9.5
  Bottom 0.152: U6.30 9.7,48.3 v20.5,37.5
RXD
  Top 0.152: S3.2 1.4,41.69 6,37.09 6,25.5 6.75,24.75 U3.18
SD_HOST_CLK  (via drill 0.2)
  Top 0.152: v23,43 21,43 15.72,48.28 U5.13
  Route2 0.152: v14,26 14,38 19,43 v23,43
  Bottom 0.152: D3.B1 14.35,25.65 v14,26 | U6.13 25.03,43 v23,43
SD_HOST_CMD  (via drill 0.2)
  Top 0.152: v11.5,37.5 11.91,37.09 U5.23 12,35.66 12,34 14.5,31.5 v14.5,26.5
  Bottom 0.152: D3.C1 14.85,26.15 v14.5,26.5 | U6.23 9.59,39.41 v11.5,37.5
SD_HOST_D0  (via drill 0.2)
  Top 0.152: v13,34 13,35.57 U5.24 13.18,37.32 v13,37.5 v13,42 | Q1.4 13.64,55.15 v13,54.5
  Route2 0.152: v13.5,25.5 13,26 v13,34 | v13,54.5 v13,42
  Bottom 0.152: v13.5,25.5 13.5,24.8 D3.A1 | U6.24 9.82,40.68 v13,37.5
SD_HOST_D1  (via drill 0.2)
  Top 0.152: v16,37.5 15.72,37.22 U5.26 15.5,35.53 v15.5,34
  Bottom 0.152: U6.26 10.28,43.22 v16,37.5 | D3.A2 12.5,25.3 12.5,31 v15.5,34
SD_HOST_D2  (via drill 0.2)
  Top 0.152: U5.14 14.5,53.2 14.5,48.5 21,42 v23,42
  Bottom 0.152: v23,42 25.2,42 U6.14 25.3,42 26.5,42 27.5,41 27.5,35.5 26.5,34.5 24,34.5 15.85,26.35 15.85,26 | 15.85,26 15.85,23.15 18,21 18,16.14 J1.1 | D2.P$1 15.85,26
SD_HOST_D3  (via drill 0.2)
  Top 0.152: U5.16 11.91,49.59 20.5,41 v23,41
  Bottom 0.152: v23,41 24.59,39.41 U6.16 23.91,39.41 23,38.5 23,35.5 15.35,27.85 D3.D1
SWDCLK  (via drill 0.2)
  Top 0.152: U2.15 18.2,6.2 19,7 21.5,7 22,7.5 v22,21.5
  Bottom 0.152: v22,21.5 23,22.5 23,24.64 J2.4
SWDIO  (via drill 0.2)
  Top 0.152: U2.16 20.8,5.5 22.52,7.22 v22.52,23
  Bottom 0.152: v22.52,23 22.52,23.85 J2.2
TXD
  Top 0.152: S3.5 6.5,40.5 6.5,26.2 U3.17
VBUS  (via drill 0.2)
  Top 0.152: R18.1 13.43,23.93 12.2,22.7 v10.7,22.7
  Bottom 0.152: U4.P$6 3.9,20.1 v5,19
  other vias: 7,21.5 7,20.5 7.5,21 8,21.5 8.5,21 8,20.5
  pour Bottom (no thermals): 6.5,26.8 6.5,20 10,20 10,26.8
  pour Route15 (no thermals): 9,7.5 4,7.5 4,19 8.5,23.5 11.5,23.5 11.5,22.3 9,22.3
VCC  (via drill 0.2)
  Top 0.152: R16.2 6.07,57.07 v6,57 | S2.1 v2,53 | U3.7 10.55,23.55 U3.6 10.25,22.25 v10.5,22
  Top 0.305: v10.5,5.5 U2.9 | v14.5,7.5 13.95,7.5 U2.F4
  Bottom 0.102: D3.B2 14.6,23.7 14.6,16.39
  Bottom 0.152: C11.P$1 19.64,23 J2.1
  Bottom 0.305: v19.5,22 19,22 C11.P$1 | v14.7,18.3 14.7,16.3 | 14.6,16.39 14.7,16.3 | 14.7,16.3 14.83,16.16 J1.4
  other vias: 7.5,32.5 8.5,32.5 8,33 9,33 30,58.5 23.5,58.5 31,51 31.5,51.5 31.5,50.5 1.5,30 1,23.5 22,58.5 22,57.5 27.5,44.5 27.5,42.5 9.5,32.5 10,33 10.5,32.5 7,33
  pour Route15 (rank 2): 0,59.5 32,59.5 32,35 23,35 23,4 0,4
  pour Bottom (no thermals): 11,33.5 6.5,33.5 6.5,29.5 11,29.5
  pour Top: 30,59.5 21.5,59.5 21.5,57 27,57 27,50 32,50 32,52 30,52
  pour Bottom: 32,58.5 27,58.5 27,58 23.5,58 23.5,58.5 21.5,58.5 21.5,57 24.5,57 24.5,55.5 29.5,55.5 29.5,51 28.5,50 28.5,47.5 27,46 27,41.5 28.5,41.5 28.5,46.5 29.5,47.5 32,47.5
  pour Top: 0,31.5 5.5,31.5 5.5,22 0,22
  pour Top: 6.5,33.5 6.5,30.5 14,30.5 14,33.5

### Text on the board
tPlace: ESP32 0 / STATUS | ESP32 0 / (FRONT) | ESP32 1 / (BACK) | nRF / STATUS | ESP32 Gateway / N. Jackson / 4/22
bPlace: ESP32 1 / STATUS
tNames: RESET | BOOT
